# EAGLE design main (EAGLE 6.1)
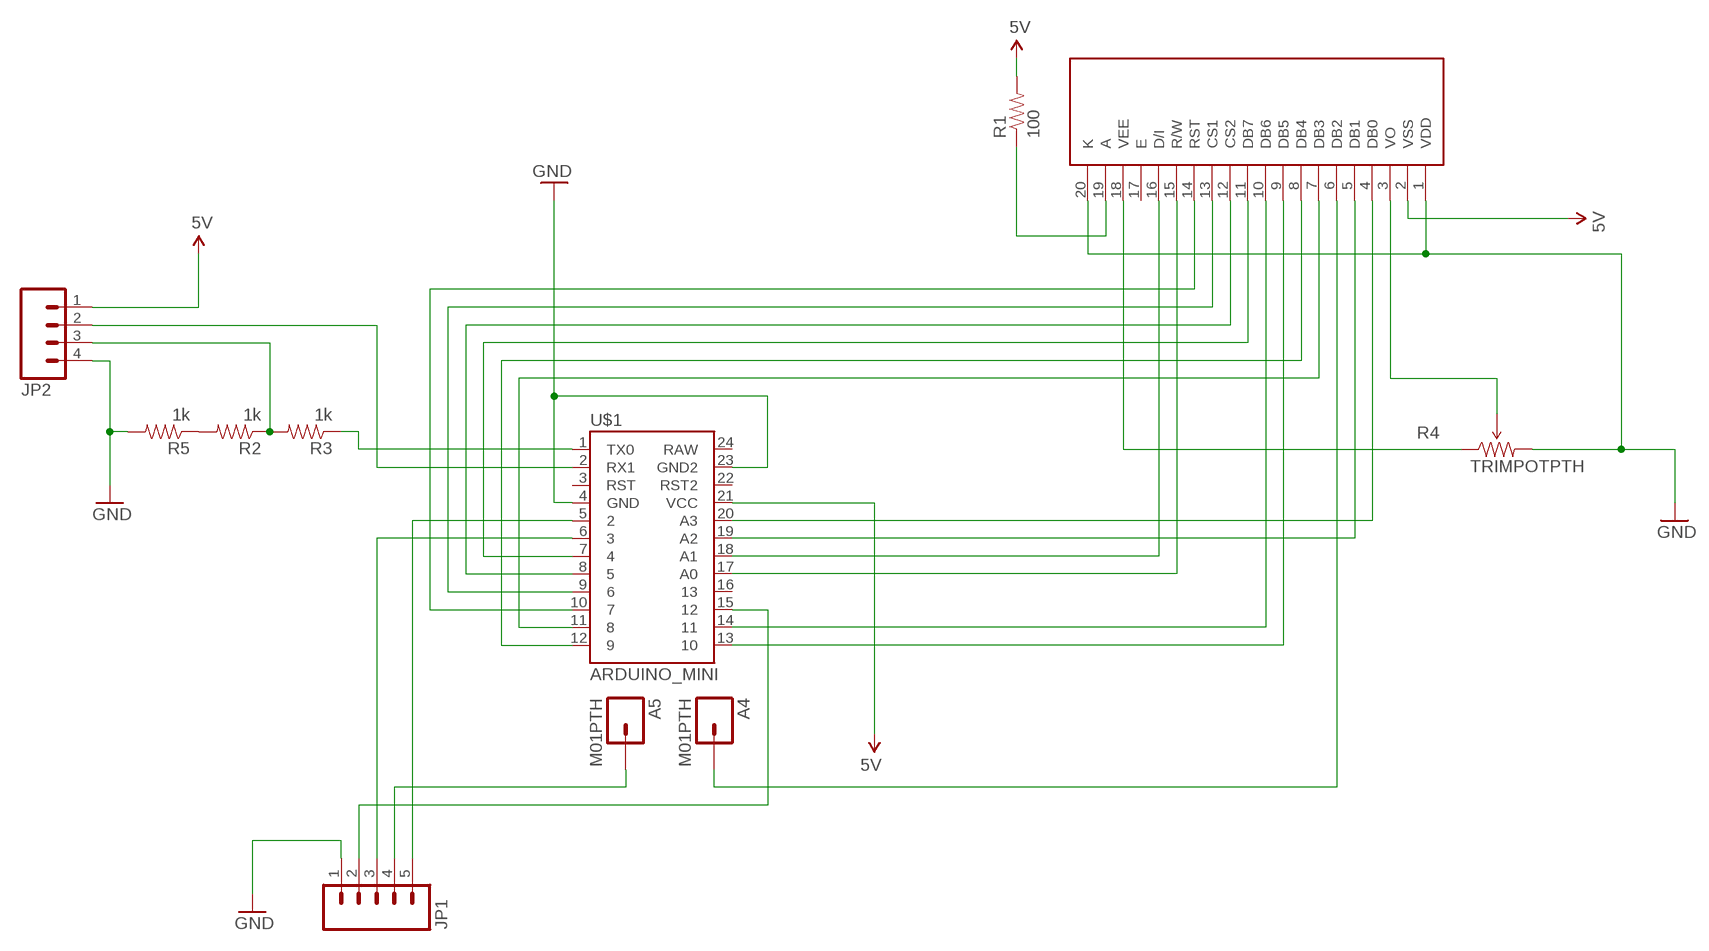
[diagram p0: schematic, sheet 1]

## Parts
A4  M01PTH  [1X01]
A5  M01PTH  [1X01]
JP1  M05PTH  [1X05]
JP2  M04PTH  [1X04]
R1  100  RESISTORPTH-1/4W  [AXIAL-0.4]
R2  1k  RESISTORPTH-1/4W  [AXIAL-0.4]
R3  1k  RESISTORPTH-1/4W  [AXIAL-0.4]
R4  TRIMPOTPTH  [TRIM_POT_PTH]
R5  1k  RESISTORPTH-1/4W  [AXIAL-0.4]
U$1  ARDUINO_MINI  [ARDUINO_MINI]
U$2  LCD-G12864BARE  [1X20]

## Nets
5V: JP2.1 R1.P$2 U$1.21(VCC) U$2.2(VSS)
GND: JP1.1 JP2.4 R4.3(CW) R5.P$2 U$1.4(GND) U$1.23(GND2) U$2.1(VDD) U$2.20(K)
N$1: R1.P$1 U$2.19(A)
N$2: U$1.20(A3) U$2.4(DB0)
N$3: U$1.19(A2) U$2.5(DB1)
N$4: U$1.11 U$2.7(DB3)
N$5: U$1.12 U$2.8(DB4)
N$6: U$1.13 U$2.9(DB5)
N$7: U$1.14 U$2.10(DB6)
N$8: U$1.7 U$2.11(DB7)
N$9: U$1.8 U$2.12(CS2)
N$10: U$1.9 U$2.13(CS1)
N$11: U$1.10 U$2.14(RST)
N$12: U$1.17(A0) U$2.15(R/W)
N$13: U$1.18(A1) U$2.16(D/I)
N$14: R4.1(CCW) U$2.18(VEE)
N$15: R4.2(WIPER) U$2.3(VO)
N$16: A4.1 U$2.6(DB2)
N$17: JP2.3 R2.P$1 R3.P$2
N$18: R3.P$1 U$1.1(TX0)
N$19: JP2.2 U$1.2(RX1)
N$20: JP1.5 U$1.5
N$21: A5.1 JP1.4
N$22: JP1.3 U$1.6
N$23: JP1.2 U$1.15
N$24: R2.P$2 R5.P$1
Unconnected: U$1.3(RST) U$1.16 U$1.22(RST2) U$1.24(RAW) U$2.17(E)

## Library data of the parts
A4 A5 = SparkFun-Connectors:M01: Header 1
JP1 = SparkFun-Connectors:M05: Header 5 Standard 5-pin 0.1" header. Use with straight break away headers (SKU : PRT-00116), right angle break away headers (PRT-00553), swiss pins (PRT-00743), machine pins (PRT-00117), and female headers (PRT-00115). Molex polarized connector foot print use with SKU : PRT-08230 with associated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
JP2 = SparkFun-Connectors:M04: Header 4 Standard 4-pin 0.1" header. Use with straight break away headers (SKU : PRT-00116), right angle break away headers (PRT-00553), swiss pins (PRT-00743), machine pins (PRT-00117), and female headers (PRT-00115). Molex polarized connector foot print use with SKU : PRT-08231 with associated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
R1-R3 R5 = SparkFun-Passives:RESISTOR: Resistor
R4 = SparkFun-Electromechanical:TRIMPOT: Various small potentiometers for "set-and-forget" applications
U$1 = SparkFun-Boards:ARDUINO_MINI: Arduino Pro Mini footprint
U$2 = SparkFun-Displays:LCD-G12864: Graphical LCD 128x64 Footprint is not yet proven. Double check it. Spark Fun Electronics SKU : LCD-00710

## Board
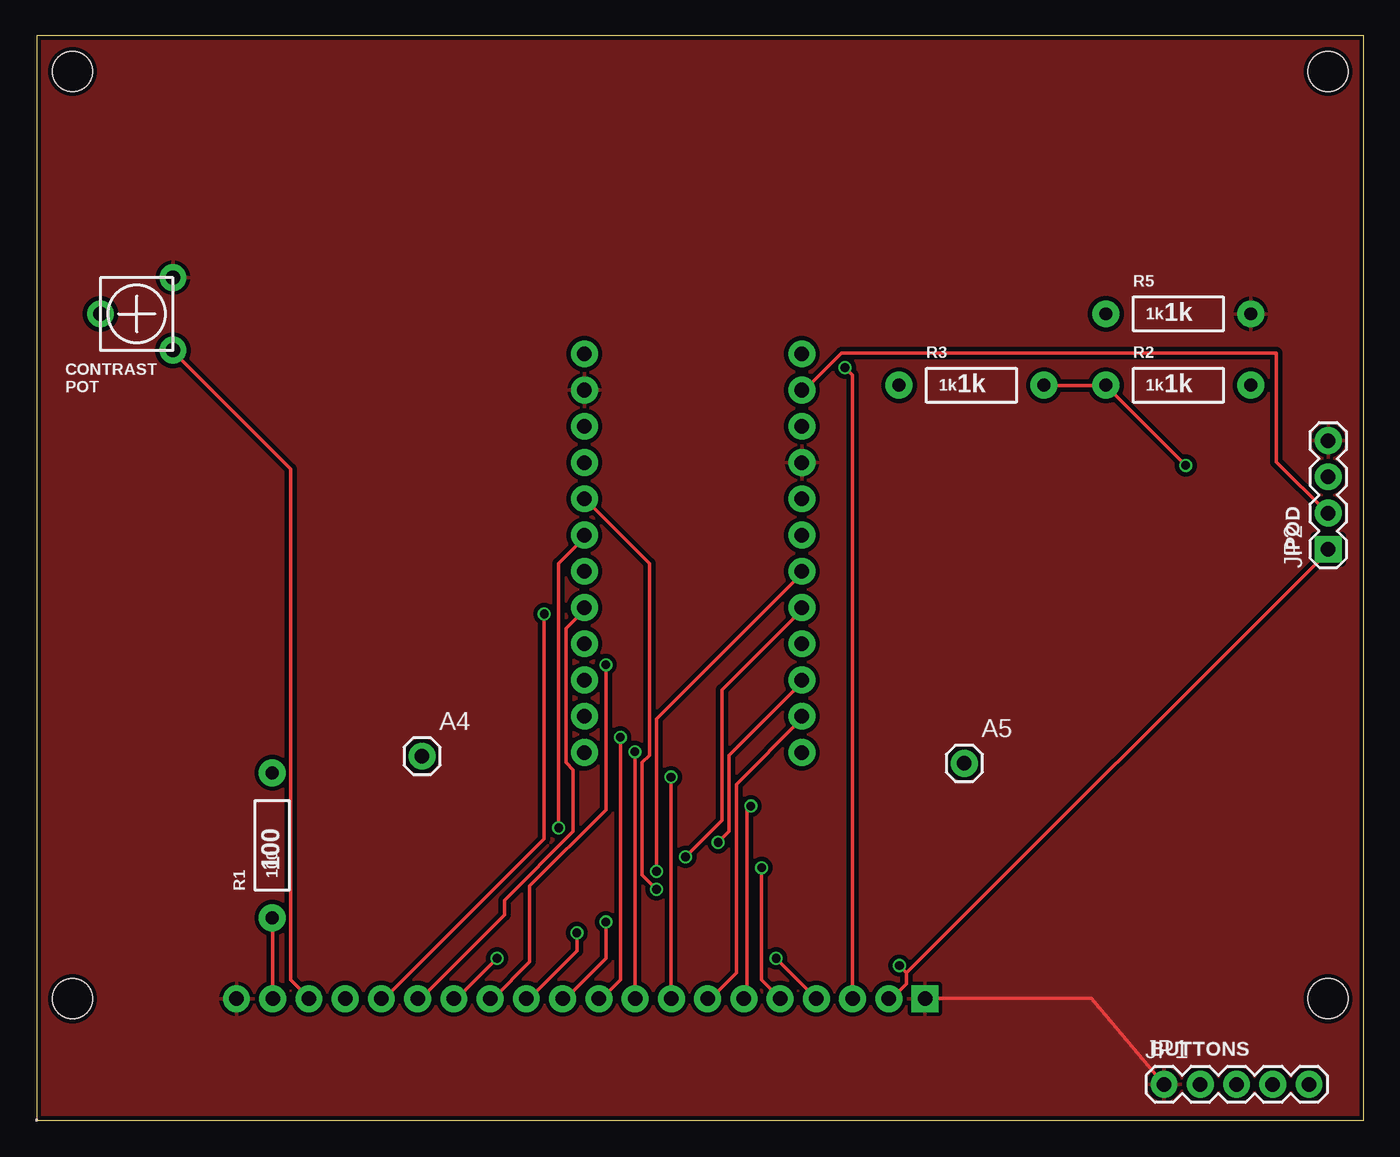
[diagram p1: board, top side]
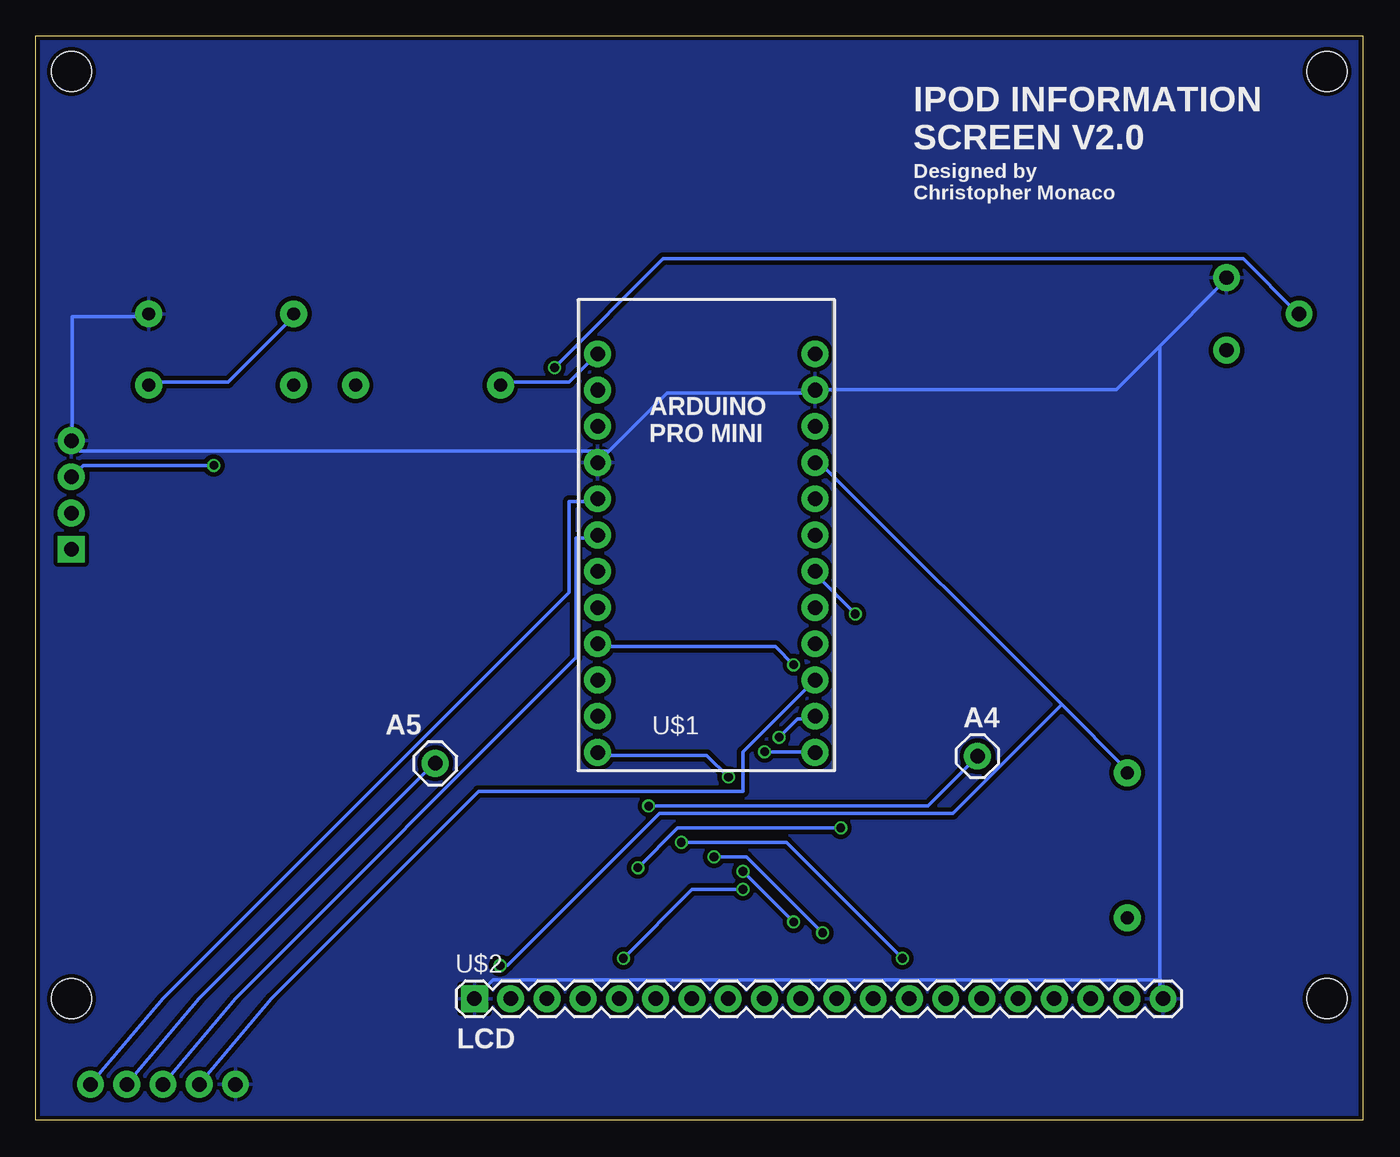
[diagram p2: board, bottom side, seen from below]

Size 93 x 76 mm. Coordinates in mm from the lower left corner, seen from the top.
Outline: 0,0 93,0 93,76 0,76 0,0
Copper layers (1*16): Top 0.035mm / dielectric 1.5mm / Bottom 0.035mm
Design rules "Fusion_eagle_rule_v1.1": minimum track width 6mil, minimum drill 12mil, track to track 6mil, track to pad 6mil, pad to pad 6mil, via to via 6mil, smd to smd 0mil, copper to edge 10mil, drill to drill 10mil, minimum pad ring 10mil, minimum via ring 6mil, stop-mask expansion 2mil, vias tented up to drill 100mil, thermal gap 10mil
Holes 2.8 mm at 2.5,8.5 2.5,73.5 90.5,73.5 90.5,8.5

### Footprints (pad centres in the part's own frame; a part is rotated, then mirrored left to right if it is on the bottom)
1X01 = drill 1.016 pad 1.88: 1 0,0
1X05 = drill 1.016 pad 1.88: 1 0,0; 2 2.54,0; 3 5.08,0; 4 7.62,0; 5 10.16,0
1X04 = drill 1.016 pad 1.88 square: 1 0,0 | drill 1.016 pad 1.88: 2 2.54,0; 3 5.08,0; 4 7.62,0
AXIAL-0.4 = drill 0.9 pad 1.88: P$1 -5.08,0; P$2 5.08,0
TRIM_POT_PTH = drill 1 pad 1.88: 1 -2.54,-2.54; 2 0,2.54; 3 2.54,-2.54
ARDUINO_MINI = drill 1.016 pad 1.88: 1 -7.62,12.7; 2 -7.62,10.16; 3 -7.62,7.62; 4 -7.62,5.08; 5 -7.62,2.54; 6 -7.62,0; 7 -7.62,-2.54; 8 -7.62,-5.08; 9 -7.62,-7.62; 10 -7.62,-10.16; 11 -7.62,-12.7; 12 -7.62,-15.24; 13 7.62,-15.24; 14 7.62,-12.7; 15 7.62,-10.16; 16 7.62,-7.62; 17 7.62,-5.08; 18 7.62,-2.54; 19 7.62,0; 20 7.62,2.54; 21 7.62,5.08; 22 7.62,7.62; 23 7.62,10.16; 24 7.62,12.7
1X20 = drill 1.016 pad 1.88 square: 1 0,0 | drill 1.016 pad 1.88: 2 2.54,0; 3 5.08,0; 4 7.62,0; 5 10.16,0; 6 12.7,0; 7 15.24,0; 8 17.78,0; 9 20.32,0; 10 22.86,0; 11 25.4,0; 12 27.94,0; 13 30.48,0; 14 33.02,0; 15 35.56,0; 16 38.1,0; 17 40.64,0; 18 43.18,0; 19 45.72,0; 20 48.26,0

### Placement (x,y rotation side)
A4  27,25.5 0 top
A5  65,25 0 top
JP1  79,2.5 0 top
JP2  90.5,40 90 top
R1  16.5,19.25 90 top
R2  80,51.5 0 top
R3  65.5,51.5 0 top
R4  7,56.5 90 top
R5  80,56.5 0 top
U$1  46,41 0 bottom
U$2  62.25,8.5 0 bottom

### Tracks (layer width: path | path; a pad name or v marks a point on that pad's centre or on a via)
5V  (via drill 0.61)
  Top 0.254: 60.96,10.32 60.96,9.56 59.94,8.54 U$2.2 | 60.96,10.32 90.42,39.78 JP2.1 | 60.96,10.32 v60.45,10.83
  Bottom 0.254: 21.08,29.11 37.85,45.88 38.35,45.88 U$1.21 | 21.08,29.11 16.51,24.54 R1.P$2 | 21.08,29.11 28.7,21.49 49.28,21.49 59.94,10.83 v60.45,10.83
GND
  Top 0.254: U$2.1 62.48,8.54 73.91,8.54 JP1.1
  Bottom 0.254: R5.P$2 85.09,56.29 90.42,56.29 90.42,47.66 JP2.4 90.42,47.4 89.92,46.89 52.83,46.89 | 14.22,54.26 17.27,51.21 38.35,51.21 U$1.23 38.61,50.96 48.77,50.96 52.83,46.89 | 14.22,54.26 9.65,58.83 R4.3 | 14.22,54.26 14.22,9.81 | 14.22,9.81 14.22,8.54 U$2.20 | 52.83,46.89 53.59,46.13 U$1.4 | 14.22,9.81 60.96,9.81 62.23,8.54 U$2.1
  pour Top (isolate 0.305): 0,0 0,76.1 92.96,76.1 92.96,0
  pour Bottom (isolate 0.305): 0,0 92.96,0 92.96,76.1 0,76.1
N$1
  Top 0.254: R1.P$1 16.51,14.13 16.51,8.54 U$2.19
N$2  (via drill 0.61)
  Top 0.254: v51.82,11.33 54.61,8.54 U$2.4 | v43.43,16.16 42.42,17.18 42.42,25.05 42.93,25.56 42.93,39.02 38.61,43.34 U$1.20
  Bottom 0.254: v51.82,11.33 46.99,16.16 v43.43,16.16
N$3  (via drill 0.61)
  Top 0.254: v50.8,17.68 50.8,9.81 52.07,8.54 U$2.5 | v36.58,20.48 36.58,39.02 38.35,40.8 U$1.19
  Bottom 0.254: v50.8,17.68 48.01,20.48 v36.58,20.48
N$4
  Top 0.254: U$2.7 47.24,8.54 49.02,10.32 49.02,23.53 53.59,28.1 U$1.11
N$5  (via drill 0.61)
  Top 0.254: v44.45,24.03 44.45,8.54 U$2.8
  Bottom 0.254: v44.45,24.03 45.97,25.56 53.59,25.56 U$1.12
N$6  (via drill 0.61)
  Top 0.254: v41.91,25.81 41.91,8.54 U$2.9
  Bottom 0.254: v41.91,25.81 38.61,25.81 U$1.13
N$7  (via drill 0.61)
  Top 0.254: v40.89,26.83 40.89,9.81 39.62,8.54 U$2.10
  Bottom 0.254: v40.89,26.83 39.62,28.1 38.61,28.1 U$1.14
N$8  (via drill 0.61)
  Top 0.254: v39.88,13.87 39.88,11.33 37.08,8.54 U$2.11 | v43.43,17.43 43.43,28.1 53.59,38.26 U$1.7
  Bottom 0.254: v43.43,17.43 v39.88,13.87
N$9  (via drill 0.61)
  Top 0.254: v37.85,13.11 37.85,11.84 34.54,8.54 U$2.12 | v45.47,18.45 48.01,20.99 48.01,30.13 53.59,35.72 U$1.8
  Bottom 0.254: v37.85,13.11 43.18,18.45 v45.47,18.45
N$10  (via drill 0.61)
  Top 0.254: v39.88,31.91 39.88,21.75 34.54,16.41 34.54,11.08 32,8.54 U$2.13
  Bottom 0.254: v39.88,31.91 41.15,33.18 53.59,33.18 U$1.9
N$11  (via drill 0.61)
  Top 0.254: v32.26,11.33 29.46,8.54 U$2.14 | v47.75,19.46 48.51,20.22 48.51,25.56 53.59,30.64 U$1.10
  Bottom 0.254: v32.26,11.33 40.39,19.46 v47.75,19.46
N$12
  Top 0.254: U$2.15 26.92,8.54 32.77,14.38 32.77,15.4 37.59,20.22 37.59,24.54 37.08,25.05 37.08,34.45 38.35,35.72 U$1.17
N$13  (via drill 0.61)
  Top 0.254: v35.56,35.46 35.56,19.72 24.38,8.54 U$2.16
  Bottom 0.254: v35.56,35.46 38.35,38.26 U$1.18
N$14
  Top 0.254: U$2.18 19.05,8.54 17.78,9.81 17.78,45.62 9.65,53.75 R4.1
N$15  (via drill 0.61)
  Top 0.254: v56.64,52.74 57.15,52.23 57.15,8.54 U$2.3
  Bottom 0.254: v56.64,52.74 49.02,60.36 8.38,60.36 4.57,56.55 R4.2
N$16  (via drill 0.61)
  Top 0.254: v50.04,22 49.78,21.75 49.78,8.54 U$2.6
  Bottom 0.254: v50.04,22 30.48,22 27.18,25.3 A4.1
N$17  (via drill 0.61)
  Top 0.254: R3.P$2 70.61,51.47 74.68,51.47 R2.P$1 74.93,51.47 v80.52,45.88
  Bottom 0.254: v80.52,45.88 89.66,45.88 90.42,45.12 JP2.3
N$18
  Bottom 0.254: U$1.1 53.85,53.5 55.63,51.72 60.2,51.72 R3.P$1
N$19
  Top 0.254: U$1.2 53.85,51.21 56.39,53.75 86.87,53.75 86.87,46.13 90.42,42.58 JP2.2
N$20
  Bottom 0.254: JP1.5 84.07,8.54 55.63,36.99 55.63,43.34 53.85,43.34 U$1.5
N$21
  Bottom 0.254: JP1.4 81.53,8.54 65.28,24.8 65.02,24.8 A5.1
N$22
  Bottom 0.254: JP1.3 78.99,8.54 55.12,32.42 55.12,40.8 53.85,40.8 U$1.6
N$23
  Bottom 0.254: U$1.15 38.61,30.64 43.43,25.81 43.43,23.02 61.98,23.02 76.45,8.54 JP1.2
N$24
  Bottom 0.254: R5.P$1 74.93,56.29 79.5,51.72 84.84,51.72 R2.P$2
N$25
  Top 0: 0,0 arc10 0,0 | 0,0 arc19 0,0 | 0,0 arc19 0,0 | 0,0 arc19 0,0 | 0,0 arc19 0,0 | 0,0 arc19 0,0 | 0,0 arc19 0,0 | 0,0 arc10 0,0 | 0,0 arc-67 0,0 | 0,0 arc10 0,0 | 0,0 | 0,0 arc19 0,0 | 0,0 | 0,0 | 0,0 | 0,0 arc19 0,0 | 0,0 | 0,0 arc19 0,0 | 0,0 | 0,0 | 0,0 | 0,0 arc19 0,0 | 0,0 | 0,0 arc19 0,0 | 0,0 | 0,0 | 0,0 | 0,0 arc19 0,0 | 0,0 | 0,0 arc10 0,0 | 0,0 | 0,0 arc-67 0,0 | 0,0 arc-248 0,0 | 0,0
N$26
  Top 0.005: 0.02,-0.05 arc10 0.03,-0.04 0.05,-0.06 0.06,-0.05 0.04,-0.03 arc19 0.05,-0.01 0.08,-0.01 0.08,0.01 0.05,0.01 arc19 0.04,0.03 0.06,0.05 0.05,0.06 0.03,0.04 arc19 0.01,0.05 0.01,0.08 -0.01,0.08 -0.01,0.05 arc19 -0.03,0.04 -0.05,0.06 -0.06,0.05 -0.04,0.03 arc19 -0.05,0.01 -0.08,0.01 -0.08,-0.01 -0.05,-0.01 arc19 -0.04,-0.03 -0.06,-0.05 -0.05,-0.06 -0.03,-0.04 arc10 -0.02,-0.05 -0.01,-0.02 arc-68 -0.02,0 arc-248 0.01,-0.02 0.02,-0.05

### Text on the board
_tsilk: 1k | CONTRAST / POT | 1k | 1k | IPOD | 100 | BUTTONS
_bsilk: IPOD INFORMATION / SCREEN V2.0 | Designed by / Christopher Monaco | ARDUINO / PRO MINI | A4 | A5 | LCD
